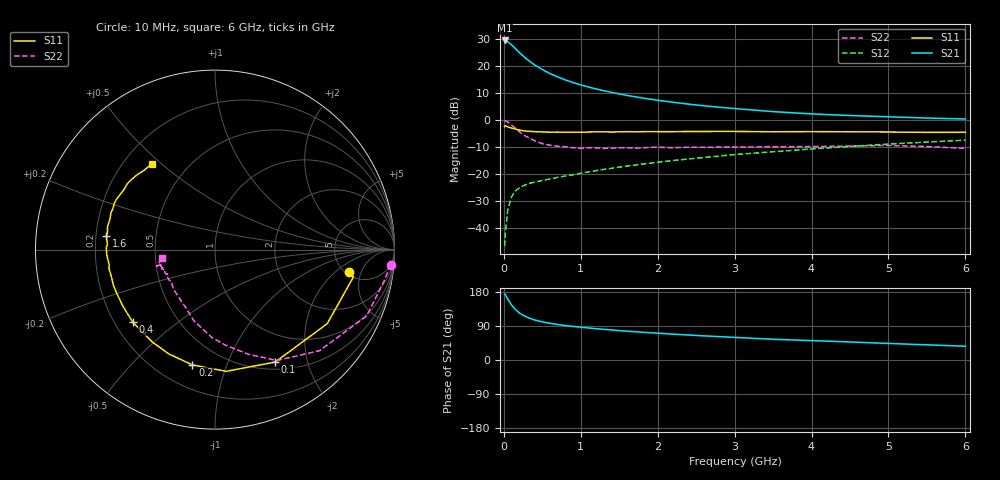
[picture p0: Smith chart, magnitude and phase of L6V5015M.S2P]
!  INFINEON TECHNOLOGIES Small Signal Semiconductors
! BFR380L3 , Si-NPN RF-Transistor in TSLP-3-1
!  Vce=0.5 V,  Ic=15 mA
! Common Emitter S-Parameters:  07. March 2005
#  GHz  S  MA  R  50
! f  S11  S21  S12  S22
! GHz  Mag  Ang  Mag  Ang  Mag  Ang  Mag  Ang
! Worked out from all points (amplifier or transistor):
!   36 points, 10 MHz to 6 GHz, reference 50 ohm
!   highest |S21| = 29.5 dB at 10 MHz (marker M1)
!   |S21| within 3 dB of that: start of sweep to 149.7 MHz
!   unconditionally stable (mu >= 1): 1.652 GHz to end of sweep
!   at 250 MHz: K = 0.35, MSG = 24.1 dB, |S12| = -24.4 dB
!   at 1.4 GHz: K = 0.97, MSG = 14.1 dB, |S12| = -17.9 dB
!   at 6 GHz: K = 1.00, MAG = 3.7 dB, |S12| = -7.4 dB
!   S11 on the Smith chart (normalised r, x): 10 MHz: 5.41, -3.17; 100 MHz: 0.59, -1.50; 200 MHz: 0.34, -0.76; 400 MHz: 0.27, -0.35; 1.6 GHz: 0.24, +0.06; 6 GHz: 0.31, +0.46
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0.01  0.7593 -9.4  29.93 174.3  0.0046 82.5  0.9814 -4.9
0.02  0.7863 -11.1  29.66 172.4  0.0082 83.9  0.9613 -9.8
0.05  0.7493 -33.4  28.38 160.9  0.0213 75.5  0.9225 -23.6
0.1  0.7108 -61.8  24.84 145.2  0.0379 62.0  0.8103 -44.0
0.15  0.681 -84.7  21.17 133.1  0.0489 54.2  0.708 -60.8
0.2  0.6547 -101.1  17.96 124.5  0.0552 49.2  0.6122 -72.3
0.25  0.6355 -113.9  15.45 118.1  0.0605 45.8  0.5356 -83.7
0.3  0.6224 -124.0  13.39 113.0  0.065 44.6  0.4901 -92.0
0.4  0.6112 -138.5  10.56 105.7  0.0708 43.5  0.4132 -106.7
0.5  0.6022 -148.3  8.651 100.7  0.0758 43.9  0.3658 -115.6
0.6  0.5994 -155.4  7.265 96.8  0.081 45.3  0.3425 -123.5
0.7  0.5999 -160.6  6.307 93.7  0.0867 46.7  0.3271 -130.6
0.9  0.6 -169.9  4.949 88.6  0.0968 49.7  0.3074 -141.1
1.1  0.6012 -175.5  4.106 84.5  0.1096 52.0  0.3073 -146.2
1.3  0.6058 179.0  3.509 80.8  0.1222 53.7  0.2981 -152.9
1.6  0.6102 172.7  2.872 76.0  0.1407 55.6  0.3067 -158.0
2.2  0.61 163.4  2.139 68.2  0.178 57.9  0.3072 -160.6
2.8  0.6179 155.0  1.732 61.7  0.2153 58.9  0.3156 -164.7
3.5  0.6076 146.6  1.435 54.7  0.2588 57.7  0.321 -164.4
4.5  0.6073 140.0  1.216 47.6  0.3252 56.3  0.3307 -164.4
5.5  0.5923 131.6  1.092 40.0  0.3915 52.4  0.3235 -166.0
6  0.5943 126.4  1.047 36.4  0.4245 50.3  0.2988 -170.7
